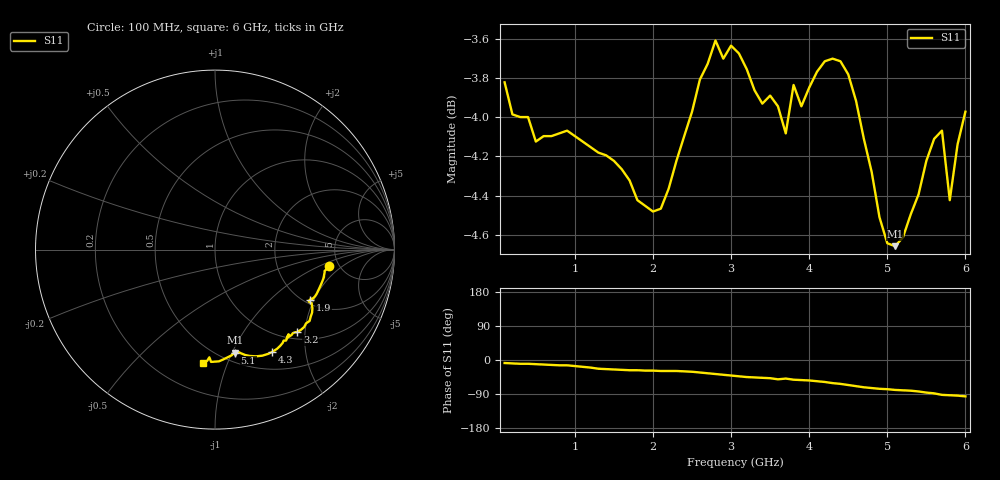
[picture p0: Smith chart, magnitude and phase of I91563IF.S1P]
!  IAM-91563  Typical Reflection Coefficients, IF port
!  Tc=25 C, Vdd= 3 V
!  LAST UPDATED 02-25-97
# ghz s ma r 50
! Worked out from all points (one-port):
!   60 points, 100 MHz to 6 GHz, reference 50 ohm
!   lowest |S11| = -4.7 dB at 5.1 GHz (marker M1), VSWR 3.82, Z = 29.4 - j51.3 ohm
!   |S11| at or under -10 dB: nowhere
!   S11 on the Smith chart (normalised r, x): 100 MHz: 4.20, -1.29; 1.9 GHz: 2.13, -1.87; 3.2 GHz: 1.15, -1.82; 4.3 GHz: 0.72, -1.44; 5.1 GHz: 0.59, -1.03; 6 GHz: 0.39, -0.82
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0.1  0.644 -8.0
0.5  0.622 -11.0
0.8  0.625 -14.0
0.9  0.626 -14.0
1.3  0.618 -23.0
1.6  0.612 -26.0
1.9  0.599 -28.0
2.1  0.598 -29.0
2.4  0.624 -30.0
2.8  0.66 -37.0
3.1  0.655 -43.0
3.2  0.649 -45.0
3.5  0.639 -48.0
3.6  0.635 -51.0
3.7  0.625 -49.0
3.8  0.643 -52.0
3.9  0.635 -53.0
4.1  0.648 -56.0
4.3  0.653 -61.0
4.4  0.652 -63.0
4.6  0.637 -69.0
4.9  0.595 -76.0
5.1  0.585 -79.0
5.3  0.596 -81.0
5.6  0.623 -88.0
5.7  0.626 -92.0
5.8  0.601 -93.0
6  0.633 -96.0
